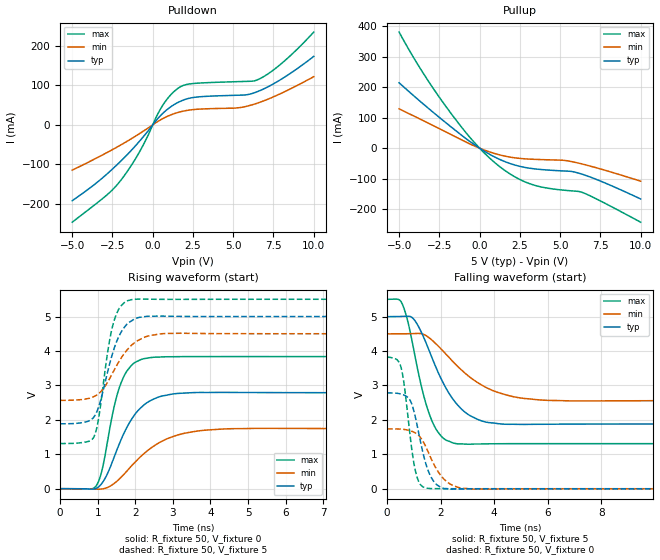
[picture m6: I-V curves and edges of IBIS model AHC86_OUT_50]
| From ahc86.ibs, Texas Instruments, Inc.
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[Model]   AHC86_OUT_50
Model_type  Output
|Vref =   0
|Rref =   1000
Cref =   50p
Vmeas =   2.5
| variable   typ   min   max
C_comp   12.39pF   11.11pF   13.60pF
| C_pullup   12.45pF   11.36pF   13.60pF
| C_pulldown   12.34pF   11.11pF   13.46pF
[Temperature Range]   40   100   -40
| Ambient temperature   25   85   -40
[Voltage range]   5   4.5   5.5
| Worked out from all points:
|   slope of the pulldown table from 0 to 0.75 V, typ, clamps not added: 22.2 ohm
|   slope of the pullup table from 0 to 0.75 V, typ, clamps not added: 31.3 ohm
|   rising waveform, R_fixture 50, V_fixture 0: 20-80 % time 733ps typ, 1.1ns min, 457ps max; typ from 0 V to 2.79 V
|   falling waveform, R_fixture 50, V_fixture 5: 20-80 % time 1.17ns typ, 1.73ns min, 753ps max; typ from 5 V to 1.88 V
|   rising waveform, R_fixture 50, V_fixture 5: 20-80 % time 482ps typ, 670ps min, 345ps max; typ from 1.88 V to 5 V
|   falling waveform, R_fixture 50, V_fixture 0: 20-80 % time 510ps typ, 714ps min, 366ps max; typ from 2.79 V to 0 V
[Pulldown]
| AHC86_OUT_50
|   Voltage   I(typ)   I(min)   I(max)
-5V       -191.8mA   -114.6mA   -246.2mA
-2.865V   -125.2mA   -70.62mA   -178mA
-2.005V   -92.58mA   -51.34mA   -141.4mA
-795mV    -40.14mA   -21.47mA   -66.35mA
560mV     26.51mA    14.37mA    45.43mA
1.005V    42.26mA    23.15mA    70.74mA
1.48V     54.77mA    30.23mA    89.72mA
2.385V    68.26mA    38.01mA    104mA
5.225V    74.86mA    42.83mA    109.2mA
6.5V      84.01mA    54.9mA     113.9mA
8.01V     116.1mA    80.32mA    155.5mA
10V       173.1mA    121.8mA    234.6mA
[Pullup]
| AHC86_OUT_50
|   Voltage   I(typ)   I(min)   I(max)
-5V       214.5mA    128.9mA    380.9mA
-3.49V    144.5mA    89.95mA    245.1mA
-1.79V    70.46mA    45.02mA    115.1mA
-235mV    8.419mA    5.273mA    13.4mA
495mV     -16.41mA   -10.12mA   -26.27mA
1.21V     -36.05mA   -21.63mA   -59.06mA
2.25V     -56.29mA   -32.15mA   -95.88mA
3.29V     -67.16mA   -36.41mA   -119.8mA
5.18V     -74.72mA   -39.75mA   -137.7mA
6.1V      -81.2mA    -48.6mA    -141.8mA
7.07V     -98.8mA    -61.76mA   -161.7mA
10V       -166.7mA   -108.3mA   -242.9mA
[Ramp]
| AHC86_OUT_50
| variable   typ   min   max
dV/dt_r   1.68/7.61E-10   1.06/1.15E-09   2.31/4.67E-10
dV/dt_f   1.88/1.20E-09   1.18/1.81E-09   2.53/7.65E-10
R_load = 50
[Rising Waveform]
| AHC86_OUT_50
R_fixture =   50
C_fixture =   0
L_fixture =   0
V_fixture =   0
V_fixture_min = 0
V_fixture_max = 0
|   Time   V(typ)   V(min)   V(max)
0s        -110.3uV   -184.5uV   -40.3uV
960ps     9.721mV    -12.7mV    84.1mV
1.23ns    370.8mV    23.13mV    1.179V
1.455ns   967.8mV    166.6mV    2.465V
1.675ns   1.558V     392.3mV    3.212V
1.985ns   2.15V      759.7mV    3.662V
2.495ns   2.605V     1.24V      3.817V
3.535ns   2.79V      1.654V     3.836V
5.22ns    2.792V     1.752V     3.837V
50ns      2.785V     1.74V      3.826V
[Falling Waveform]
| AHC86_OUT_50
R_fixture =   50
C_fixture =   0
L_fixture =   0
V_fixture =   5
V_fixture_min = 4.5
V_fixture_max = 5.5
|   Time   V(typ)   V(min)   V(max)
0s        5V         4.5V       5.502V
550ps     5.007V     4.501V     5.398V
1.02ns    4.907V     4.509V     3.951V
1.38ns    4.38V      4.48V      2.675V
1.73ns    3.708V     4.281V     1.881V
2.115ns   3.048V     3.982V     1.461V
2.625ns   2.444V     3.565V     1.306V
3.7ns     1.936V     2.943V     1.304V
6.085ns   1.874V     2.565V     1.31V
50ns      1.884V     2.564V     1.311V
[Rising Waveform]
| AHC86_OUT_50
R_fixture =   50
C_fixture =   0
L_fixture =   0
V_fixture =   5
V_fixture_min = 4.5
V_fixture_max = 5.5
|   Time   V(typ)   V(min)   V(max)
0s        1.884V     2.564V     1.311V
890ps     2.071V     2.671V     1.486V
1.015ns   2.346V     2.752V     1.99V
1.275ns   3.442V     3.116V     4.043V
1.43ns    4.05V      3.429V     4.858V
1.62ns    4.542V     3.788V     5.31V
1.965ns   4.918V     4.227V     5.501V
2.39ns    5.011V     4.447V     5.503V
3.205ns   5.003V     4.514V     5.498V
50ns      5V         4.5V       5.502V
[Falling Waveform]
| AHC86_OUT_50
R_fixture =   50
C_fixture =   0
L_fixture =   0
V_fixture =   0
V_fixture_min = 0
V_fixture_max = 0
|   Time   V(typ)   V(min)   V(max)
0s        2.785V     1.74V      3.826V
515ps     2.752V     1.731V     3.547V
650ps     2.718V     1.721V     2.966V
865ps     2.565V     1.686V     1.523V
1.015ns   2.219V     1.639V     693.1mV
1.155ns   1.725V     1.568V     261.8mV
1.575ns   450.1mV    1.001V     8.452mV
2.265ns   -3.032mV   185.2mV    1.277mV
3.26ns    -665.3uV   -11.61mV   -156.9uV
50ns      -110.3uV   -184.4uV   -40.32uV
